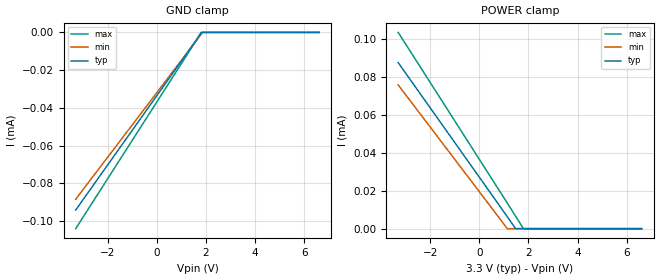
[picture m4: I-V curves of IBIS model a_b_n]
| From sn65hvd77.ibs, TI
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[Model]   a_b_n
Model_type   Input
Vinl = 0.8
Vinh = 2
|   typ   min   max
|   (nom PVT)   (fast PVT)   (slow PVT)
|Average
C_comp   3.329e-12   3.222e-12   3.479e-12
| Where nom  PVT is Nominal Process, 3.3V, 27C
|   Fast PVT is Strong Process,  3.6V, -40C
|   Slow PVT is Weak Process,   3V, 150C
[Voltage Range]   3.3   3   3.6
|Ambient Temperature   25   125   -40
|Junction Temperature
[Temperature Range]   27   150   -40
[Power Clamp Reference]   3.3   3   3.6
[GND Clamp Reference]   0   0   0
[GND Clamp]
|   Voltage   I(typ)   I(min)   I(max)
-3.3V     -94.06uA   -88.34uA   -103.9uA
1.805V    -328.5nA   -972.3nA   -24.74nA
1.866V    0A         0A         0A
6.6V      0A         0A         0A
[POWER Clamp]
|   Voltage   I(typ)   I(min)   I(max)
-3.3V     87.76uA    75.97uA    103.7uA
1.137V    6.303uA    27.73nA    13.52uA
1.475V    43.76nA    0A         6.596uA
1.794V    0A         0A         0A
6.6V      0A         0A         0A
